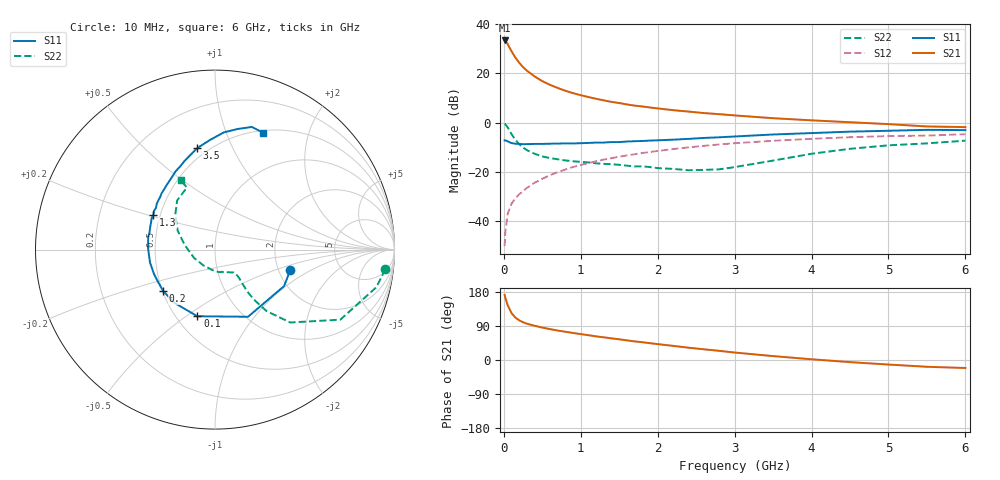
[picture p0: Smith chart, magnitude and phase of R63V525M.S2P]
! SIEMENS Small Signal Semiconductors
! BFR193
! Si NPN RF Bipolar Junction Transistor in SOT23
! VCE = 3.5 V  IC = 25 mA
! Common Emitter S-Parameters:  May  1996
# GHz  S  MA  R  50
!  f  S11  S21  S12  S22
! GHz  MAG  ANG  MAG  ANG  MAG  ANG  MAG  ANG
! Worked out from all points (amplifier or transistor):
!   36 points, 10 MHz to 6 GHz, reference 50 ohm
!   highest |S21| = 33.4 dB at 10 MHz (marker M1)
!   |S21| within 3 dB of that: start of sweep to 76.01 MHz
!   unconditionally stable (mu >= 1): 497.3 MHz to 1.963 GHz
!   at 250 MHz: K = 0.88, MSG = 25.2 dB, |S12| = -27.8 dB
!   at 1.4 GHz: K = 1.02, MAG = 10.5 dB, |S12| = -14.4 dB
!   at 6 GHz: K = 0.95, MSG = 1.4 dB, |S12| = -4.7 dB
!   S11 on the Smith chart (normalised r, x): 10 MHz: 2.33, -0.64; 100 MHz: 0.63, -0.55; 200 MHz: 0.50, -0.27; 1.3 GHz: 0.46, +0.21; 3.5 GHz: 0.44, +0.74; 6 GHz: 0.52, +1.36
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0.01  0.4348 -14.8  46.6 171.8  0.0031 87.3  0.9553 -6.6
0.02  0.4354 -27.8  45.2 164.0  0.0061 80.3  0.9233 -13.1
0.05  0.4171 -63.8  39.16 144.5  0.014 70.6  0.8 -29.2
0.1  0.3841 -104.8  28.16 123.8  0.0227 66.2  0.5837 -44.1
0.15  0.373 -127.2  20.87 111.9  0.029 64.4  0.4474 -50.0
0.2  0.3696 -141.2  16.44 104.7  0.0351 65.8  0.3649 -51.8
0.25  0.3648 -151.0  13.4 99.6  0.0407 66.7  0.3116 -52.4
0.3  0.3661 -158.2  11.33 95.8  0.0473 68.6  0.2759 -52.0
0.4  0.3692 -168.7  8.665 90.3  0.0601 69.9  0.2331 -50.8
0.5  0.3693 -176.0  6.96 85.6  0.0725 70.2  0.2059 -49.6
0.6  0.3733 178.3  5.852 81.5  0.0857 70.5  0.1904 -49.4
0.7  0.3752 173.2  5.057 77.7  0.0986 70.4  0.1802 -49.9
0.8  0.3789 169.1  4.433 74.5  0.1119 69.5  0.1706 -50.3
0.9  0.3771 165.2  3.966 71.3  0.1253 68.5  0.1639 -51.0
1.1  0.387 157.1  3.303 65.4  0.1513 66.9  0.1555 -55.2
1.3  0.3941 150.5  2.828 59.8  0.1775 64.5  0.1454 -59.8
1.7  0.4191 138.5  2.215 49.1  0.228 59.4  0.1293 -72.9
2.2  0.4508 126.3  1.79 37.3  0.2904 52.4  0.1149 -98.2
3.5  0.5741 99.9  1.229 10.3  0.4278 32.6  0.1696 171.9
4.5  0.6554 85.6  1.018 -5.6  0.5056 18.4  0.2938 138.9
5.5  0.7135 73.3  0.836 -17.9  0.5453 4.1  0.3792 114.4
6  0.7048 67.7  0.811 -21.1  0.5815 0.1  0.4303 116.1
